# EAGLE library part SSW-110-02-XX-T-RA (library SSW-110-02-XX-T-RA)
30 Position Receptacle Connector Through Hole, Right Angle Check prices
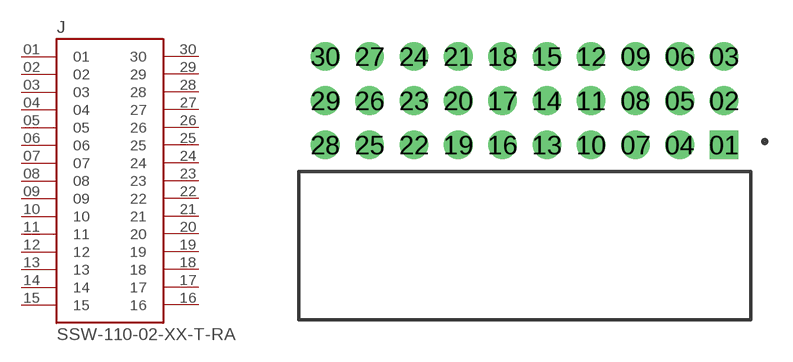
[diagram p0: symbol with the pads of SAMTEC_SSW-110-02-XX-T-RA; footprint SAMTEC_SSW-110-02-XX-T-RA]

Designator prefix J

## SSW-110-02-XX-T-RAJ (Availability: Bad; Description: CONN RCPT 30POS 0.1 GOLD PCB R/A; MF: Samtec; MP: SSW-110-02-L-T-RA; Package: None; Price: None; Purchase-URL: https://pricing.snapeda.com/search/part/SSW-110-02-L-T-RA/?ref=eda)  [SAMTEC_SSW-110-02-XX-T-RA]
01  01  pas
02  02  pas
03  03  pas
04  04  pas
05  05  pas
06  06  pas
07  07  pas
08  08  pas
09  09  pas
10  10  pas
11  11  pas
12  12  pas
13  13  pas
14  14  pas
15  15  pas
16  16  pas
17  17  pas
18  18  pas
19  19  pas
20  20  pas
21  21  pas
22  22  pas
23  23  pas
24  24  pas
25  25  pas
26  26  pas
27  27  pas
28  28  pas
29  29  pas
30  30  pas

## Footprint SAMTEC_SSW-110-02-XX-T-RA (pad centres in mm)
translated Allegro footprint
drill 1.04 pad 1.64 square: 01 11.43,0
drill 1.04 pad 1.64: 02 11.43,2.54; 03 11.43,5.08; 04 8.89,0; 05 8.89,2.54; 06 8.89,5.08; 07 6.35,0; 08 6.35,2.54; 09 6.35,5.08; 10 3.81,0; 11 3.81,2.54; 12 3.81,5.08; 13 1.27,0; 14 1.27,2.54; 15 1.27,5.08; 16 -1.27,0; 17 -1.27,2.54; 18 -1.27,5.08; 19 -3.81,0; 20 -3.81,2.54; 21 -3.81,5.08; 22 -6.35,0; 23 -6.35,2.54; 24 -6.35,5.08; 25 -8.89,0; 26 -8.89,2.54; 27 -8.89,5.08; 28 -11.43,0; 29 -11.43,2.54; 30 -11.43,5.08

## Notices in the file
This work is licensed under a Creative Commons Attribution-ShareAlike 4.0 International License (CC BY-SA) with Design Exception 1.0
